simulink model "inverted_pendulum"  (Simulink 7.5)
settings: Solver=ode45  StartTime=0.0  StopTime=inf  RelTol=1e-3
libraries: simulink x2, simulink_extras x1

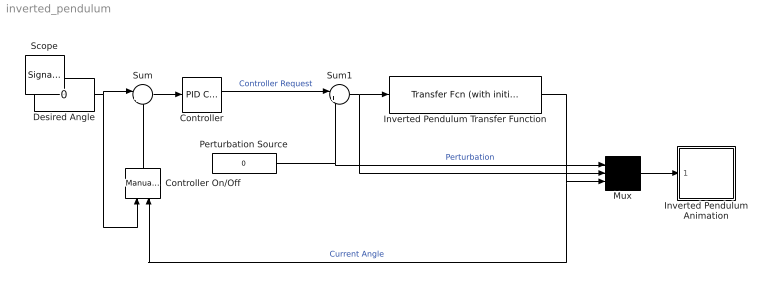
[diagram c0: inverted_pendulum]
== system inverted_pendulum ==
  Controller : simulink/Continuous/PID Controller  DialogController=pidpack.PIDConfig.pidDDGCreate  DialogControllerArgs=DataTag0  SystemSampleTime=-1  Controller=PID  TimeDomain=Continuous-time  SampleTime=1  IntegratorMethod=Forward Euler  FilterMethod=Forward Euler  Form=Parallel  P=8.58883340676243  I=4.57247198874764  D=2.23434739173045  N=765.110458624984  InitialConditionSource=internal  InitialConditionForIntegrator=0  InitialConditionForFilter=0  ExternalReset=none  LimitOutput=off  UpperSaturationLimit=10  LowerSaturationLimit=-10  LinearizeAsGain=off  AntiWindupMode=none  Kb=1  TrackingMode=off  Kt=1  PParamMin=[]  PParamMax=[]  IParamMin=[]  IParamMax=[]  DParamMin=[]  DParamMax=[]  NParamMin=[]  NParamMax=[]  KbParamMin=[]  KbParamMax=[]  KtParamMin=[]  KtParamMax=[]  POutMin=[]  POutMax=[]  IOutMin=[]  IOutMax=[]  DOutMin=[]  DOutMax=[]  NOutMin=[]  NOutMax=[]  KbOutMin=[]  KbOutMax=[]  KtOutMin=[]  KtOutMax=[]  IntegratorOutMin=[]  IntegratorOutMax=[]  FilterOutMin=[]  FilterOutMax=[]  SumOutMin=[]  SumOutMax=[]  SumI1OutMin=[]  SumI1OutMax=[]  SumI2OutMin=[]  SumI2OutMax=[]  SumI3OutMin=[]  SumI3OutMax=[]  SumDOutMin=[]  SumDOutMax=[]  SaturationOutMin=[]  SaturationOutMax=[]  IntegratorContinuousStateAttributes=''  IntegratorStateMustResolveToSignalObject=off  IntegratorRTWStateStorageClass=Auto  FilterContinuousStateAttributes=''  FilterStateMustResolveToSignalObject=off  FilterRTWStateStorageClass=Auto
  Controller On/Off : simulink/Signal Routing/Manual Switch  SystemSampleTime=-1  sw=0  action=0  varsize=off
  Desired Angle : Constant  Value=0  OutDataType=fixdt(1, 16)  OutScaling=2^0
  Inverted Pendulum Animation : Subsystem  mask(Pendulum plot){RefBlock=Perturbation Source}
      mask prompts: RefBlock "DC reference signal block name:"
      mask help: Pendulum plot
  Inverted Pendulum Transfer Function : simulink_extras/Additional Linear/Transfer Fcn (with initial states)  SystemSampleTime=-1  N=[4.545 0]  D=[1 0.1818 -31.18 -4.455]  X0=0
  Mux : Mux  Inputs=3
  Perturbation Source : Constant  Value=0  OutDataType=fixdt(1, 16)  OutScaling=2^0
  Sum : Sum  Inputs=|+-  OutDataType=fixdt(1, 16)  OutScaling=2^0
  Sum1 : Sum  Inputs=|++  OutDataType=fixdt(1, 16)  OutScaling=2^0
  Scope : SignalViewerScope  IOType=viewer  NumInputPorts=3  RefreshTime=0.035000
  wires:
  Inverted Pendulum Transfer Function/1 -> Controller On/Off/2, Mux/3  "Current Angle"
  Sum/1 -> Controller/1
  Desired Angle/1 -> Sum/1, Controller On/Off/1
  Controller On/Off/1 -> Sum/2
  Mux/1 -> Inverted Pendulum Animation/1(in_1)
  Sum1/1 -> Inverted Pendulum Transfer Function/1, Mux/2
  Perturbation Source/1 -> Sum1/2, Mux/1  "Perturbation"
  Controller/1 -> Sum1/1  "Controller Request"

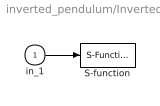
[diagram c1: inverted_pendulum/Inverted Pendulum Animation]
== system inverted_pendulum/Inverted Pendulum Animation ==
  in_1 : Inport  OutDataType=sfix(16)  OutScaling=2^0
  S-function : S-Function  FunctionName=pendan  Parameters=RefBlock  EnableBusSupport=off
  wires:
  in_1/1 -> S-function/1
